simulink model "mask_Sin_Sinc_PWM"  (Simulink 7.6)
settings: Solver=ode15s  StartTime=0.0  StopTime=N  RelTol=1e-3
InitFcn:
  | N=100
StopFcn:
  | clc
  | load SortieGenerateur.mat
  | plot(x(1,:),x(2,:))
  | xlabel('temps')
  | title('Signal de sortie du générateur de signaux')
  | grid
undefined symbols (not defined in the file or in its folder): Sinusoïde
libraries: nesl_utility x1

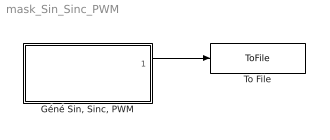
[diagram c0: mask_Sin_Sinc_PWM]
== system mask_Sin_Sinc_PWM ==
  "Géné Sin, Sinc, PWM" : Subsystem  mask(Masque de générateur de signaux (sinus, sinus cardinal, PWM)){f=1/20, Ampl=5, ChoixSignal=Sinusoïde, PWM=off, rc=80}
      mask prompts: f "fréquence :"; Ampl "amplitude:"; PWM "Signal PWM"; rc "Rapport Cyclique [0 ... 100]"
      mask help: Masque générateur de 3 signaux: - sinusoïde - sinus cardinal - signal PWM
      mask init:
      | switch ChoixSignal
      | case 1, % Sinus
      |        str='sin';
      |        x=-pi:pi/100:pi;
      |        y=sin(x);
      |        rc=80;
      | case 2, % Sinc
      |        str='sinc';
      |        x=-pi:pi/100:pi;
      |        y=sinc(x);
      | end
      | 
      | parametres=get_param(gcb,'MaskValues');
      | p4=parametres{4}; 
      | if strcmp(p4,'on'); 
      |     str='PWM';
      |     x=0:0.01:10;
      |     y=square(x,70);
      | end
  To File : ToFile  Filename=SortieGenerateur  MatrixName=x
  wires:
  "Géné Sin, Sinc, PWM"/1(S) -> To File/1

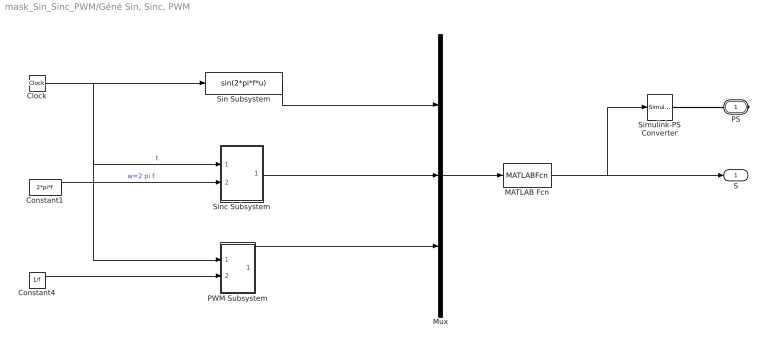
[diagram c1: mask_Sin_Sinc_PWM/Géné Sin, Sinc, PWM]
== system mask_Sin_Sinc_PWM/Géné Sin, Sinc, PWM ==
  Clock : Clock
  Constant1 : Constant  Value=2*pi*f
  Constant4 : Constant  Value=1/f
  MATLAB Fcn : MATLABFcn  MATLABFcn=((ChoixSignal==1) && (PWM~=1))*u(1)+((ChoixSignal==2) && (PWM~=1))*u(2)+(PWM==1) *u(3)
  Mux : Mux  Inputs=3
  PWM Subsystem : Subsystem
  Simulink-PS Converter : nesl_utility/Simulink-PS Converter  DialogController=NetworkEngine.DynNeUtilDlgSource  SystemSampleTime=-1  PhysicalDomain=network_engine_domain  LeftPortType=input  RightPortType=output  SubClassName=ps_input  Unit=1  AffineConversion=off  InputFilterTimeConstant=.001  UdotUserProvided=0
  Sin Subsystem : Fcn  Expr=sin(2*pi*f*u)
  Sinc Subsystem : Subsystem
  PS : PMIOPort  Tag=PMCPort  Port=1  Side=Right
  S : Outport
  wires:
  Clock/1 -> Sinc Subsystem/1(t), PWM Subsystem/1(t), Sin Subsystem/1  "t"
  Constant1/1 -> Sinc Subsystem/2(w)  "w=2 pi f"
  Constant4/1 -> PWM Subsystem/2(T)
  PWM Subsystem/1(PWM) -> Mux/3
  Mux/1 -> MATLAB Fcn/1
  MATLAB Fcn/1 -> S/1, Simulink-PS Converter/1
  Sin Subsystem/1 -> Mux/1
  Sinc Subsystem/1(sinc) -> Mux/2
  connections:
  Simulink-PS Converter/RConn1 -- PS/RConn1

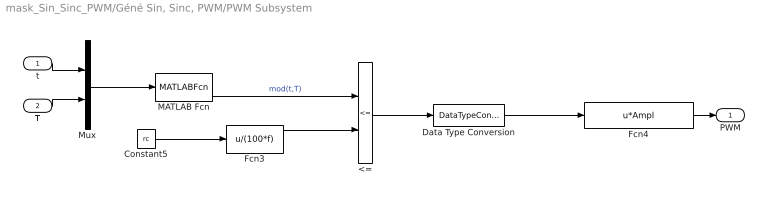
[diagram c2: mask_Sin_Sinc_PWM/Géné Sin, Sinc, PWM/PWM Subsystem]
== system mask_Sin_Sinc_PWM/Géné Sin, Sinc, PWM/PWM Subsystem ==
  t : Inport
  T : Inport  Port=2
  <= : RelationalOperator  Operator=<=
  Constant5 : Constant  Value=rc
  Data Type Conversion : DataTypeConversion  OutDataTypeStr=double
  Fcn3 : Fcn  Expr=u/(100*f)
  Fcn4 : Fcn  Expr=u*Ampl
  MATLAB Fcn : MATLABFcn  MATLABFcn=mod(u(1),u(2))  OutputDimensions=1
  Mux : Mux  Inputs=2
  PWM : Outport
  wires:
  Mux/1 -> MATLAB Fcn/1
  Constant5/1 -> Fcn3/1
  MATLAB Fcn/1 -> <=/1  "mod(t,T)"
  Fcn3/1 -> <=/2
  <=/1 -> Data Type Conversion/1
  Data Type Conversion/1 -> Fcn4/1
  t/1 -> Mux/1
  T/1 -> Mux/2
  Fcn4/1 -> PWM/1

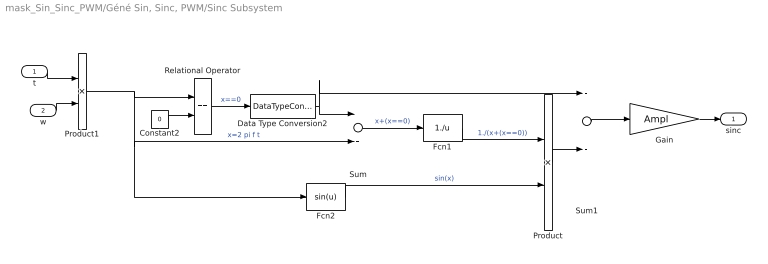
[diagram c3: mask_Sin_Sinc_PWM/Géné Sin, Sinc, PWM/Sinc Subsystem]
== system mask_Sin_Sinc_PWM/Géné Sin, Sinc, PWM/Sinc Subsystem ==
  t : Inport
  w : Inport  Port=2
  Constant2 : Constant  Value=0
  Data Type Conversion2 : DataTypeConversion  OutDataTypeStr=double
  Fcn1 : Fcn  Expr=1./u
  Fcn2 : Fcn  Expr=sin(u)
  Gain : Gain  Gain=Ampl
  Product : Product
  Product1 : Product
  Relational Operator : RelationalOperator  Operator===
  Sum : Sum
  Sum1 : Sum
  sinc : Outport
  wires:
  Sum1/1 -> Gain/1
  Product/1 -> Sum1/2
  Relational Operator/1 -> Data Type Conversion2/1  "x==0"
  Sum/1 -> Fcn1/1  "x+(x==0)"
  Product1/1 -> Fcn2/1, Sum/2, Relational Operator/1  "x=2 pi f t"
  Fcn2/1 -> Product/2  "sin(x)"
  Fcn1/1 -> Product/1  "1./(x+(x==0))"
  Constant2/1 -> Relational Operator/2
  Data Type Conversion2/1 -> Sum1/1, Sum/1
  t/1 -> Product1/1
  w/1 -> Product1/2
  Gain/1 -> sinc/1
